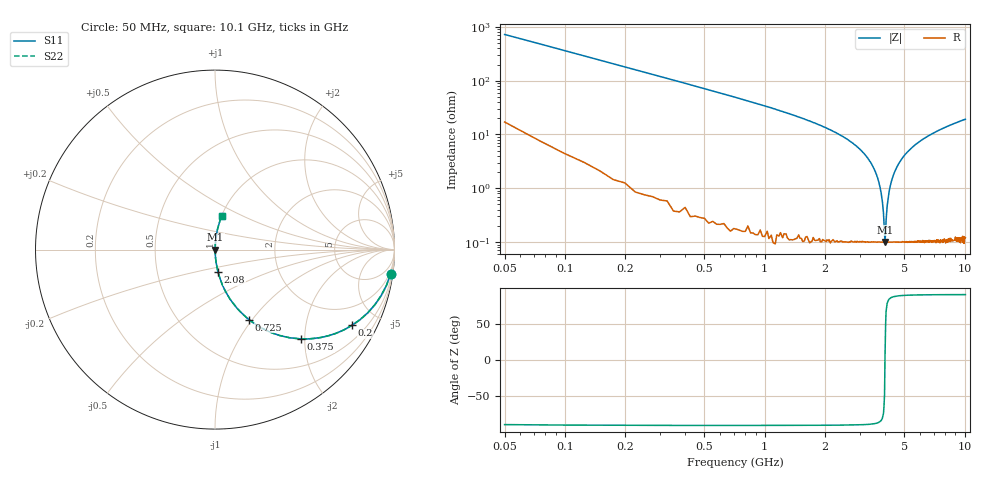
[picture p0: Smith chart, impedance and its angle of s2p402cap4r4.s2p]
! AVX Thin Film Operation		Date: April 2003
! Description: Accu-P® Series, Thin Film, SMD, RF Capacitor
! Part Number: 04025J4R4ABS
! 50 MHz  -  10.05 GHz
! Serial Measurements
# hz S db R 50
!	S11		S21		S12		S22
!	dB	Phase	dB	Phase	dB	Phase	dB	Phase
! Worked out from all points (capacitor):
!   400 points, 50 MHz to 10.1 GHz, reference 50 ohm
!   read as one part in series: C = 4.4 pF near 100 MHz
!   lowest |Z| = 100 mohm at 4 GHz (marker M1)
!   series resonance near 3.999 GHz, so ESL is about 360 pH
!   S11 on the Smith chart (normalised r, x): 50 MHz: 1, -14; 200 MHz: 1.03, -3.61; 375 MHz: 1.01, -1.91; 725 MHz: 1.00, -0.96; 2.08 GHz: 1.00, -0.25; 10.1 GHz: 1.00, +0.38
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5e7  -0.11 -7.8  -17.30 80.8  -17.30 80.8  -0.11 -7.8
1e8  -0.35 -15.4  -11.50 73.9  -11.50 73.9  -0.35 -15.4
2e8  -1.19 -28.9  -6.31 60.7  -6.31 60.7  -1.19 -28.9
3.75e8  -3.23 -46.2  -2.84 43.6  -2.84 43.6  -3.23 -46.2
7.25e8  -7.25 -64.1  -0.92 25.7  -0.92 25.7  -7.25 -64.1
1.73e9  -15.50 -80.0  -0.13 9.7  -0.13 9.7  -15.50 -80.0
2.08e9  -18.00 -82.3  -0.08 7.2  -0.08 7.2  -18.00 -82.3
2.88e9  -24.30 -85.6  -0.02 3.5  -0.02 3.5  -24.30 -85.6
3.4e9  -30.60 -86.4  -0.01 1.7  -0.01 1.7  -30.60 -86.4
3.68e9  -36.30 -85.4  -0.01 0.9  -0.01 0.9  -36.30 -85.4
3.83e9  -41.80 -82.5  -0.01 0.5  -0.01 0.5  -41.80 -82.5
3.93e9  -49.10 -73.3  -0.01 0.2  -0.01 0.2  -49.10 -73.3
4e9  -60.00 2.8  -0.01 -0.0  -0.01 -0.0  -60.00 2.8
4.03e9  -56.20 49.6  -0.01 -0.1  -0.01 -0.1  -56.20 49.6
4.05e9  -52.00 66.3  -0.01 -0.1  -0.01 -0.1  -52.00 66.3
4.1e9  -46.70 77.3  -0.01 -0.3  -0.01 -0.3  -46.70 77.3
4.25e9  -39.10 84.2  -0.01 -0.6  -0.01 -0.6  -39.10 84.2
4.55e9  -32.60 86.2  -0.01 -1.3  -0.01 -1.3  -32.60 86.2
5.08e9  -27.20 86.2  -0.02 -2.5  -0.02 -2.5  -27.20 86.2
6.75e9  -20.10 83.7  -0.05 -5.7  -0.05 -5.7  -20.10 83.7
8.43e9  -16.70 81.2  -0.10 -8.4  -0.10 -8.4  -16.70 81.2
1.01e10  -14.50 78.8  -0.17 -10.8  -0.17 -10.8  -14.50 78.8
